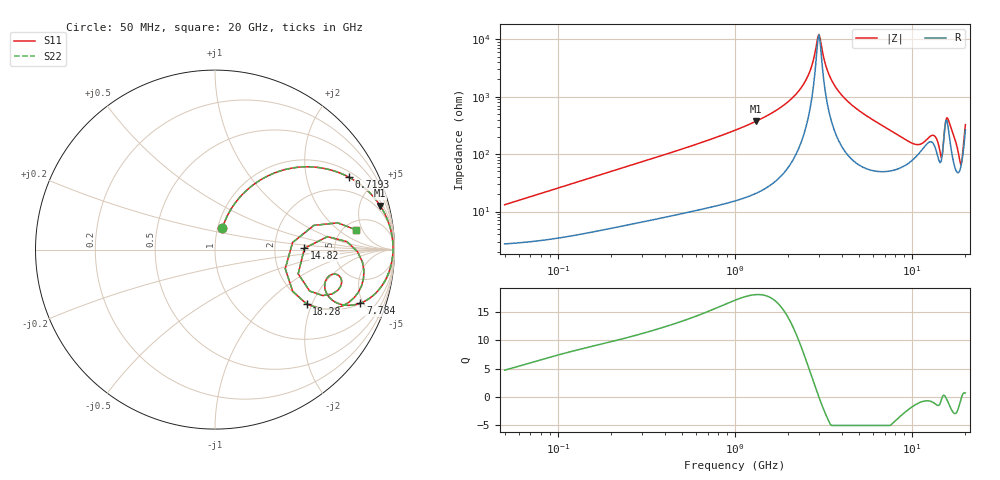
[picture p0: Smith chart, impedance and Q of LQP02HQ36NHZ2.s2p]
!Murata Part Number: LQP02HQ36NHZ2
!These Parameters are Measured in Series Mode Connection
!  o--[Z]--o
!Port1  Port2
!  o-------o
!Freq. Start=50[MHz] Stop=20[GHz], 401[Steps]
# Hz S RI R 50
!Freq.(Hz) S11(Real) S11(Imag) S21(Real) S21(Imag) S12(Real) S12(Imag) S22(Real) S22(Imag)
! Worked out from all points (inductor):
!   401 points, 50 MHz to 20 GHz, reference 50 ohm
!   read as one part in series: L = 40.7 nH near 51.52 MHz
!   highest Q = 18 at 1.309 GHz (marker M1), where L = 45.1 nH
!   self-resonance near 2.94 GHz
!   S11 on the Smith chart (normalised r, x): 50 MHz: 1.05, +0.26; 719.3 MHz: 1.24, +3.56; 7.784 GHz: 2.04, -4.77; 14.82 GHz: 2.99, +0.06; 18.28 GHz: 1.95, -1.83; 20 GHz: 6.33, +3.76
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5e7  0.0415 0.1198  0.9585 -0.1198  0.9585 -0.1198  0.0415 0.1198
1.364002e8  0.133 0.2855  0.867 -0.2855  0.867 -0.2855  0.133 0.2855
3.721004e8  0.4561 0.4581  0.5439 -0.4581  0.5439 -0.4581  0.4561 0.4581
7.192613e8  0.7471 0.4029  0.2529 -0.4029  0.2529 -0.4029  0.7471 0.4029
1e9  0.8571 0.3217  0.1429 -0.3217  0.1429 -0.3217  0.8571 0.3217
1.309461e9  0.9206 0.2439  0.0794 -0.2439  0.0794 -0.2439  0.9206 0.2439
2.146657e9  0.9823 0.0966  0.0177 -0.0966  0.0177 -0.0966  0.9823 0.0966
2.728004e9  0.9915 0.0258  0.00847 -0.0258  0.00847 -0.0258  0.9915 0.0258
2.98453e9  0.9919 -0.00081  0.00815 0.00081  0.00815 0.00081  0.9919 -0.00081
3.364474e9  0.9895 -0.0367  0.0105 0.0367  0.0105 0.0367  0.9895 -0.0367
3.908127e9  0.9817 -0.0826  0.0183 0.0826  0.0183 0.0826  0.9817 -0.0826
7.442007e9  0.8335 -0.2879  0.1665 0.2879  0.1665 0.2879  0.8335 -0.2879
7.784049e9  0.8099 -0.2983  0.1901 0.2983  0.1901 0.2983  0.8099 -0.2983
1.019291e10  0.6309 -0.2586  0.3691 0.2586  0.3691 0.2586  0.6309 -0.2586
1.220001e10  0.6602 -0.1367  0.3398 0.1367  0.3398 0.1367  0.6602 -0.1367
1.396067e10  0.6525 -0.2474  0.3475 0.2474  0.3475 0.2474  0.6525 -0.2474
1.482269e10  0.4984 0.00776  0.5016 -0.00776  0.5016 -0.00776  0.4984 0.00776
1.597544e10  0.8297 -0.1184  0.1703 0.1184  0.1703 0.1184  0.8297 -0.1184
1.747767e10  0.7055 -0.3166  0.2945 0.3166  0.2945 0.3166  0.7055 -0.3166
1.828096e10  0.5102 -0.3035  0.4898 0.3035  0.4898 0.3035  0.5102 -0.3035
1.88369e10  0.3914 -0.1064  0.6086 0.1064  0.6086 0.1064  0.3914 -0.1064
2e10  0.7841 0.1107  0.2159 -0.1107  0.2159 -0.1107  0.7841 0.1107
